FUNCTION_BLOCK FB_LN_IED_LD1_LEDGGIO8 EXTENDS FB_AcsiCommonLogicalNodeClass
VAR_INPUT
	NamPlt: FB_DO_IED_LD1_LEDGGIO8_NamPlt := (sClass:='LPL', bLinkResult:=THIS^.AddDataToContainer(ipData:=NamPlt));
	Beh: FB_DO_IED_LD1_LEDGGIO8_Beh := (sClass:='ENS', bLinkResult:=THIS^.AddDataToContainer(ipData:=Beh));
	Health: FB_DO_IED_LD1_LEDGGIO8_Health := (sClass:='ENS', bLinkResult:=THIS^.AddDataToContainer(ipData:=Health));
	Mod_: FB_DO_IED_LD1_LEDGGIO8_Mod := (sObjectName:='Mod', sClass:='ENC', bLinkResult:=THIS^.AddDataToContainer(ipData:=Mod_));
	SPCSO1: FB_DO_IED_LD1_LEDGGIO8_SPCSO1 := (sClass:='SPC', bLinkResult:=THIS^.AddDataToContainer(ipData:=SPCSO1));
END_VAR
VAR
END_VAR

END_FUNCTION_BLOCK
